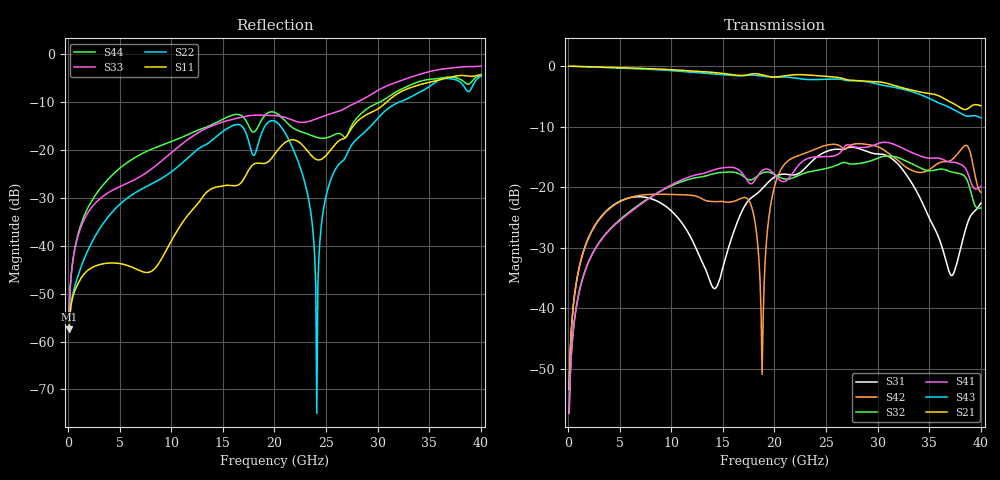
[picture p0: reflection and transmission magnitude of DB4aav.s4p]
! ADC12DJ2700AAV, ADC12DJ3200AAV, ADC08DJ3200AAV
! 144 pin AAV package
! Texas Instruments 4/21/2021
! Single-ended  S-parameters
! PORT#  PORT_NAME  NET_NAME
! PORT1:  DAxN.DIEBUMP DAxN
! PORT2:  DAxN.BGA  DAxN
! PORT3:  DAxP.DIEBUMP DAxP
! PORT4:  DAxP.BGA  DAxP
! Touchstone Ver. 1.0
! Number of ports is 4
# Hz	S	MA	R	50.000000
! SCATTERING PARAMETERS  :
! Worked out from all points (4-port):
!   400 points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, 100 MHz to 40 GHz, reference 50 ohm
!   strongest paths, dB at 100 MHz, 10.1 GHz, 20.1 GHz, 30.1 GHz, 40 GHz:
!     S21: 0.0, -0.6, -1.8, -2.6, -6.6
!     S43: 0.0, -0.8, -1.8, -3.0, -8.5
!     S41: -57.4, -19.5, -18.1, -12.8, -19.9
!     S32: -57.4, -19.7, -18.0, -15.2, -23.4
!     S42: -53.4, -21.2, -19.3, -13.4, -20.9
!     S31: -53.4, -24.1, -18.2, -14.5, -22.6
!   lowest |S11| = -57.5 dB at 100 MHz (marker M1), VSWR 1.00, Z = 50.1 + j0.0766 ohm
!   |S11| at or under -10 dB: start of sweep to 30.86 GHz
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1e8  0.001336 34.9  0.9987 -1.0  0.002135 85.5  0.001354 -96.2
     0.9987 -1.0  0.001345 34.0  0.001354 -96.2  0.002133 85.3
     0.002135 85.5  0.001354 -96.2  0.002048 60.2  0.9988 -1.0
     0.001354 -96.2  0.002133 85.3  0.9988 -1.0  0.002058 59.0
1.88e10  0.07231 -5.1  0.847 -175.9  0.09691 78.5  0.1369 63.8
         0.847 -175.9  0.1544 -96.6  0.1309 61.2  0.002841 114.7
         0.09691 78.5  0.1309 61.2  0.2308 10.2  0.8264 -168.2
         0.1369 63.8  0.002841 114.7  0.8264 -168.2  0.2096 -125.2
2e10  0.09001 -1.9  0.8126 174.8  0.1212 69.2  0.1274 43.2
      0.8126 174.8  0.2003 -132.2  0.1273 44.2  0.1008 150.4
      0.1212 69.2  0.1273 44.2  0.2286 3.3  0.8137 -178.1
      0.1274 43.2  0.1008 150.4  0.8137 -178.1  0.2474 -155.2
2.35e10  0.0894 -46.4  0.8417 140.7  0.16 57.5  0.1754 24.8
         0.8417 140.7  0.02299 171.0  0.1346 22.4  0.1989 54.9
         0.16 57.5  0.1346 22.4  0.2014 2.7  0.7732 150.6
         0.1754 24.8  0.1989 54.9  0.7732 150.6  0.1431 133.2
2.41e10  0.0793 -37.9  0.8343 134.5  0.1775 52.6  0.1778 16.4
         0.8343 134.5  0.000178 -127.0  0.1376 16.8  0.2089 45.5
         0.1775 52.6  0.1376 16.8  0.2125 3.8  0.774 145.6
         0.1778 16.4  0.2089 45.5  0.774 145.6  0.1354 112.4
2.58e10  0.1116 -16.4  0.8123 116.9  0.205 34.4  0.1817 -0.5
         0.8123 116.9  0.05986 -28.0  0.1493 1.6  0.226 17.6
         0.205 34.4  0.1493 1.6  0.246 3.5  0.7819 129.4
         0.1817 -0.5  0.226 17.6  0.7819 129.4  0.1444 45.0
4e10  0.6123 -132.0  0.4696 -20.9  0.07386 123.9  0.1012 -172.0
      0.4696 -20.9  0.5917 -97.4  0.06747 -152.8  0.09053 89.2
      0.07386 123.9  0.06747 -152.8  0.7504 -89.0  0.3743 -5.4
      0.1012 -172.0  0.09053 89.2  0.3743 -5.4  0.5961 -112.7
